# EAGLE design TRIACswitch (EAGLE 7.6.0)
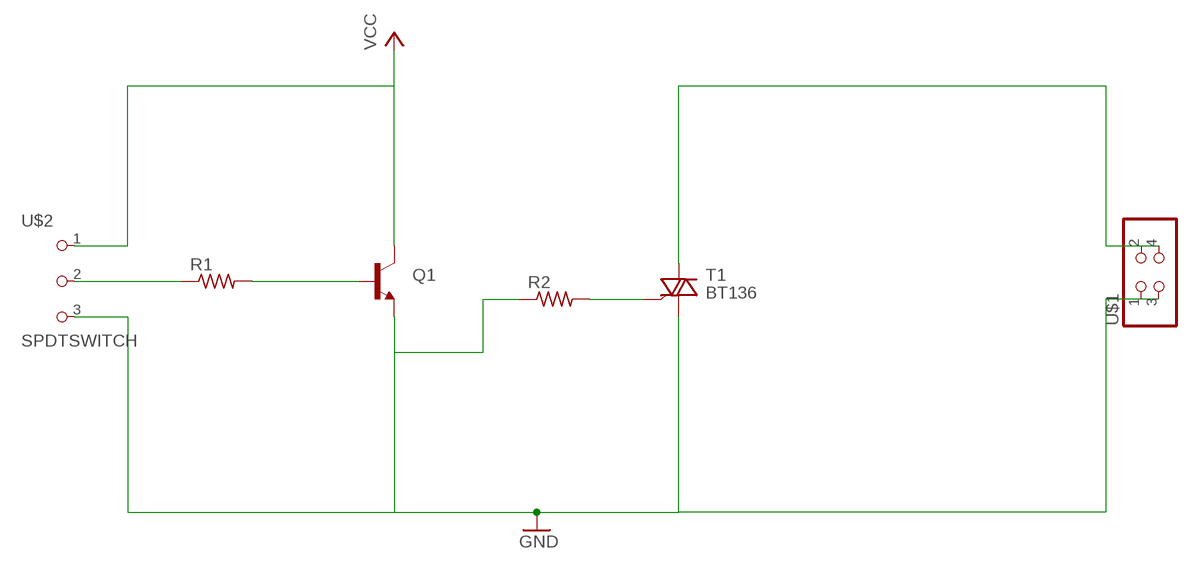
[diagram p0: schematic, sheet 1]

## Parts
Q1  TRANSISTOR_NPNBC547  [TO-92-AMMO]
R1  RES-US1206FAB  [R1206FAB]
R2  RES-US1206FAB  [R1206FAB]
T1  BT136  [TO220AB]
U$1  PINHD-2X2-SMD  [2X02SMD]
U$2  SPDTSWITCH  [SPDTSWITCH]

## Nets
GND: Q1.3(E) R2.1 T1.1(A1) U$1.3 U$2.3
N$2: R1.1 U$2.2
N$3: Q1.2(B) R1.2
N$4: R2.2 T1.3(G)
N$6: T1.2(A2) U$1.4
VCC: Q1.1(C) U$2.1
Unconnected: U$1.1 U$1.2

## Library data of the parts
Q1 = SparkFun-DiscreteSemi:TRANSISTOR_NPN: Generic NPN BJT MMBT2222A - TRANS-08049 (SOT-23, 1A 40V) MPSA42 - TRANS-09116 (SOT-23, 500mA 300V) MMBT5088LT1G - TRANS-11160 (SOT-23, 50 mA 30V) BC547 - COM-08928 (TO-92 45V 100mA) (1.Collector 2.Base 3.Emitter) 2N3904 - COM-00521 (TO-92 40V 200mA) (1.Emitter 2.Base 3.Collector) P2N2222A -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
R1 R2 = fab:RES-US: Resistor (US Symbol)
T1 = triac:BT136: Triac BT136 series E sensitive gate Source: http://www.nxp.com/acrobat_download/datasheets/BT136_SERIES_E_2.pdf
U$1 = fab:PINHD-2X2-SMD
U$2 = fab:SPDTSWITCH

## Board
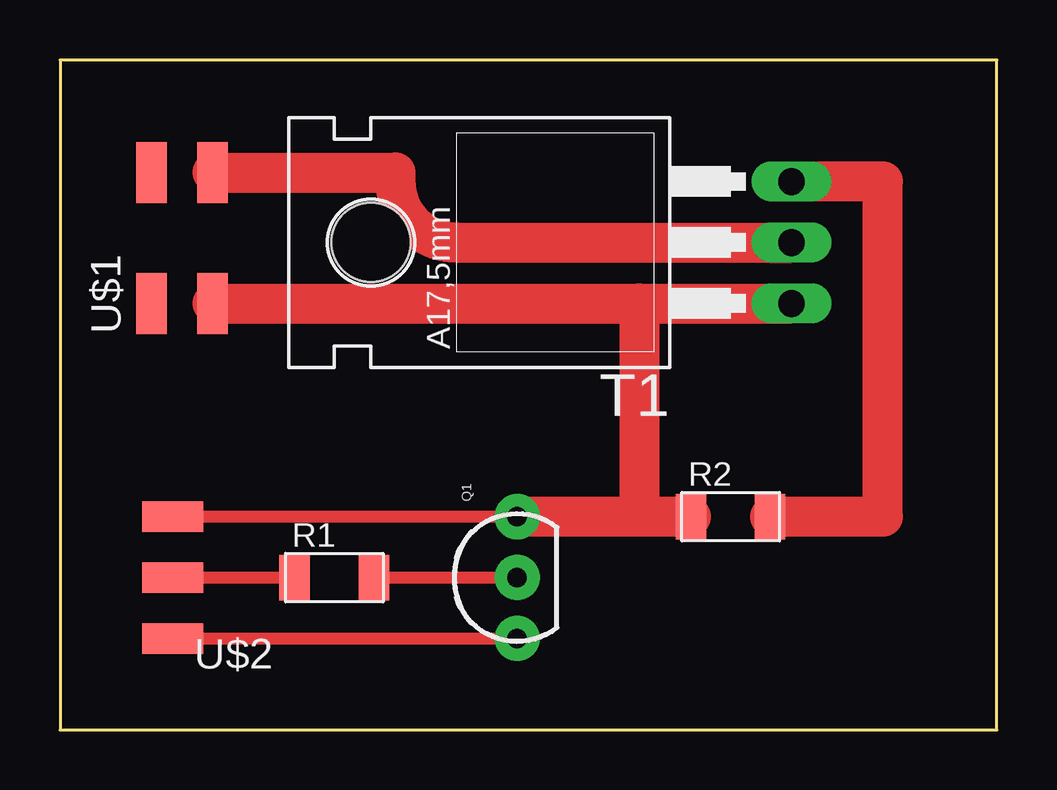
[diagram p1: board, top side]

Size 39.04 x 27.93 mm. Coordinates in mm from the lower left corner, seen from the top.
Outline: 0,0 39.04,0 39.04,27.93 0,27.93 0,0
Copper layers (1*16): Top 0.035mm / dielectric 1.5mm / Bottom 0.035mm
Design rules "default *": minimum track width 18mil, minimum drill 24mil, track to track 16mil, track to pad 16mil, pad to pad 16mil, via to via 16mil, smd to smd 8mil, copper to edge 40mil, drill to drill 8mil, minimum pad ring 10mil, minimum via ring 8mil, stop-mask expansion 4mil, vias tented up to drill 0mil, thermal gap 10mil

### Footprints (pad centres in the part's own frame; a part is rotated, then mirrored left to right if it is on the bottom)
TO-92-AMMO = drill 0.813 pad 1.88: 1 -2.54,0; 2 0,0; 3 2.54,0
R1206FAB = smd 1.27 x 1.905: 1 -1.651,0; 2 1.651,0
TO220AB = drill 1.118 long: 1 -2.54,-6.35; 2 0,-6.35; 3 2.54,-6.35 | hole 3.302: 0,11.176
2X02SMD = smd 2.54 x 1.27: 1 -2.54,1.27; 2 2.92,1.27; 3 -2.54,-1.27; 4 2.92,-1.27
SPDTSWITCH = smd 2.54 x 1.27: 1 0.38,2.54; 2 0.38,0; 3 0.38,-2.54

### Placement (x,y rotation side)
Q1  19.05,6.35 90 top
R1  11.43,6.35 0 top
R2  27.94,8.89 0 top
T1  24.13,20.32 90 top
U$1  5.08,20.32 90 top
U$2  5.08,6.35 180 top

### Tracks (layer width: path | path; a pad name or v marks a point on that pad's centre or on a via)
GND
  Top 0.508: U$2.3 Q1.3
  Top 1.676: T1.1 U$1.3 24.13,17.78 24.13,8.89 | Q1.3 24.13,8.89 | 24.13,8.89 R2.1
N$2
  Top 0.508: U$2.2 R1.1
N$3
  Top 0.508: R1.2 Q1.2
N$4
  Top 0.508: 34.29,22.86 34.29,9.78
  Top 1.676: R2.2 34.29,8.89 34.29,22.86 T1.3
N$6
  Top 1.676: U$1.4 13.97,23.24 13.97,22.86 arc90 16.51,20.32 T1.2
VCC
  Top 0.508: U$2.1 Q1.1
